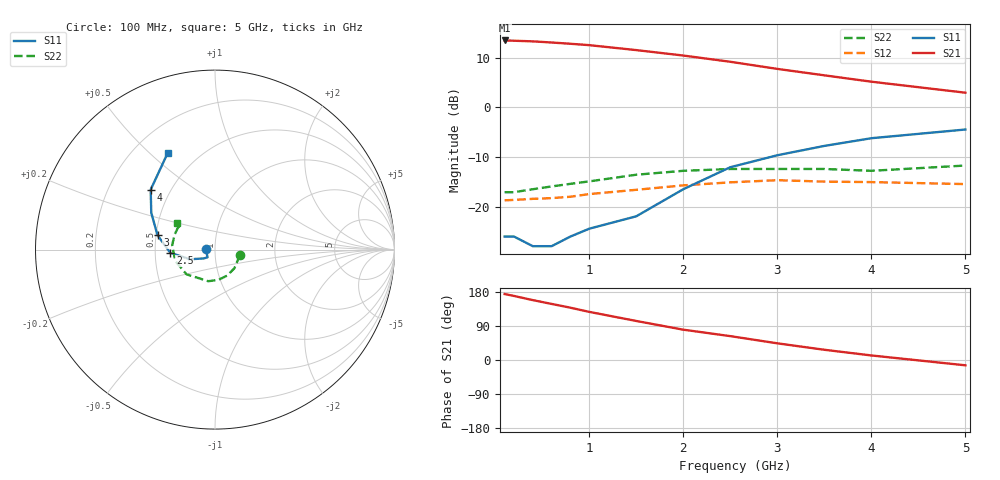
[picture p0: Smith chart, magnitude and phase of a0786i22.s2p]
!  MSA-0786 S AND NOISE PARAMETERS
!  Id=22mA  LAST UPDATED 07-27-92
# ghz s ma r 50
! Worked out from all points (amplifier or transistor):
!   13 points, 100 MHz to 5 GHz, reference 50 ohm
!   highest |S21| = 13.5 dB at 100 MHz (marker M1)
!   |S21| within 3 dB of that: start of sweep to 1.981 GHz
!   unconditionally stable (mu >= 1): start of sweep to end of sweep
!   at 400 MHz: K = 1.15, MAG = 13.5 dB, |S12| = -18.4 dB
!   at 1.5 GHz: K = 1.11, MAG = 12.0 dB, |S12| = -16.6 dB
!   at 5 GHz: K = 1.32, MAG = 5.8 dB, |S12| = -15.4 dB
!   lowest NFmin = 4.80 dB at 100 MHz
!   S11 on the Smith chart (normalised r, x): 100 MHz: 0.91, +0.01; 2.5 GHz: 0.60, -0.02; 3 GHz: 0.51, +0.09; 4 GHz: 0.39, +0.34; 5 GHz: 0.34, +0.57
0.1  0.05 175.0  4.74 174.0  0.116 1.0  0.14 -12.0
0.2  0.05 174.0  4.71 169.0  0.117 3.0  0.14 -22.0
0.4  0.04 167.0  4.64 158.0  0.12 4.0  0.15 -44.0
0.6  0.04 175.0  4.52 148.0  0.122 7.0  0.16 -65.0
0.8  0.05 -158.0  4.39 138.0  0.126 8.0  0.17 -84.0
1  0.06 -134.0  4.25 127.0  0.134 10.0  0.18 -102.0
1.5  0.08 -142.0  3.79 103.0  0.148 9.0  0.21 -139.0
2  0.15 -159.0  3.34 80.0  0.164 7.0  0.23 -164.0
2.5  0.25 -176.0  2.89 63.0  0.176 5.0  0.24 174.0
3  0.33 166.0  2.45 44.0  0.185 1.0  0.24 159.0
3.5  0.41 150.0  2.11 27.0  0.179 -5.0  0.24 149.0
4  0.49 137.0  1.82 12.0  0.177 -9.0  0.23 145.0
5  0.6 116.0  1.41 -14.0  0.169 -14.0  0.26 145.0
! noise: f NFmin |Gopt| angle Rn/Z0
0.1  4.8  0.06  0  0.61
0.5  4.9  0.05  -2  0.6
1  5  0.04  -12  0.59
2  5.6  0.07  -101  0.57
